FUNCTION_BLOCK Resume_DUT

VAR_IN_OUT
    SD_SMD_IO: DUT_AMCI_Stepper;
END_VAR	

VAR_INPUT
			
END_VAR

VAR_OUTPUT
	Enable: BOOL;
	Error: BOOL; 
END_VAR

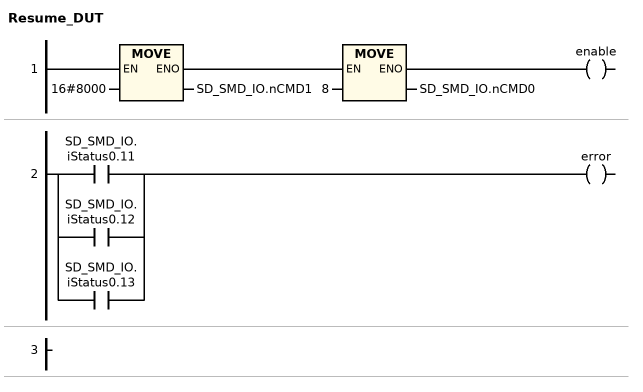
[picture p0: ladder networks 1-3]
// NETWORK 1
SD_SMD_IO.nCMD1 := 16#8000;
SD_SMD_IO.nCMD0 := 8;
enable := TRUE;

// NETWORK 2
error := SD_SMD_IO.iStatus0.11 OR SD_SMD_IO.iStatus0.12 OR SD_SMD_IO.iStatus0.13;

// NETWORK 3

END_FUNCTION_BLOCK
